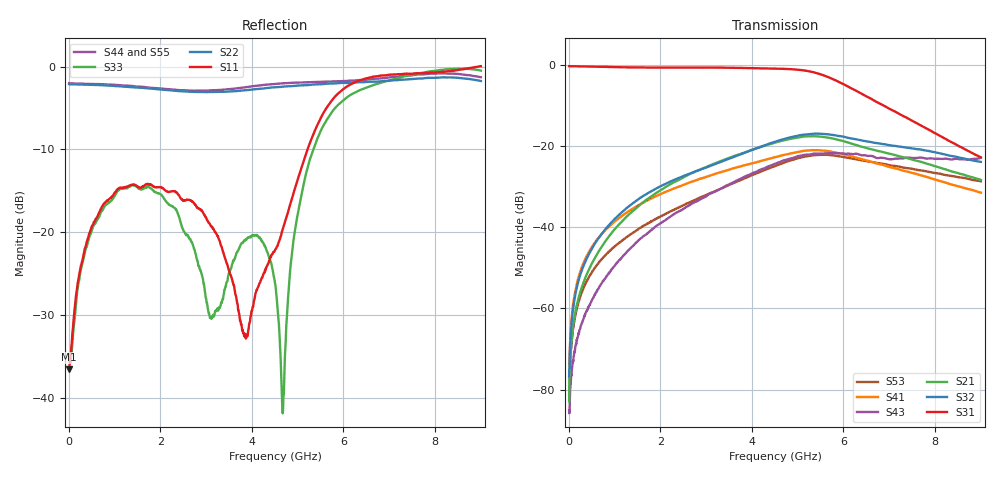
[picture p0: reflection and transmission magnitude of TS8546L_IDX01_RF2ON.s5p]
# GHz S DB R 50
! CMT, SN0916, 25263762, 26.7.0
! Date: 16.07.2026 12:21:51
! Data: Format
! Freq S1.1:dB/Ang S1.2:dB/Ang S1.3:dB/Ang S1.4:dB/Ang S1.5:dB/Ang
!  S2.1:dB/Ang S2.2:dB/Ang S2.3:dB/Ang S2.4:dB/Ang S2.5:dB/Ang
!  S3.1:dB/Ang S3.2:dB/Ang S3.3:dB/Ang S3.4:dB/Ang S3.5:dB/Ang
!  S4.1:dB/Ang S4.2:dB/Ang S4.3:dB/Ang S4.4:dB/Ang S4.5:dB/Ang
!  S5.1:dB/Ang S5.2:dB/Ang S5.3:dB/Ang S5.4:dB/Ang S5.5:dB/Ang
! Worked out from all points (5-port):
!   2001 points, 10 MHz to 9 GHz, reference 50 ohm
!   strongest paths, dB at 10 MHz, 2.257 GHz, 4.505 GHz, 6.753 GHz, 9 GHz:
!     S31: -0.2, -0.5, -0.8, -9.2, -22.7
!     S32: -76.7, -28.5, -18.9, -19.2, -23.8
!     S21: -82.9, -29.1, -19.1, -21.1, -28.3
!     S43: -85.1, -37.0, -24.3, -22.9, -22.9
!     S41: -77.5, -30.6, -22.6, -24.3, -31.4
!     S53: -81.1, -35.8, -24.8, -24.1, -28.6
!   lowest |S11| = -36.6 dB at 10 MHz (marker M1), VSWR 1.03, Z = 51.5 - j0.0982 ohm
!   |S11| at or under -10 dB: start of sweep to 5.216 GHz
